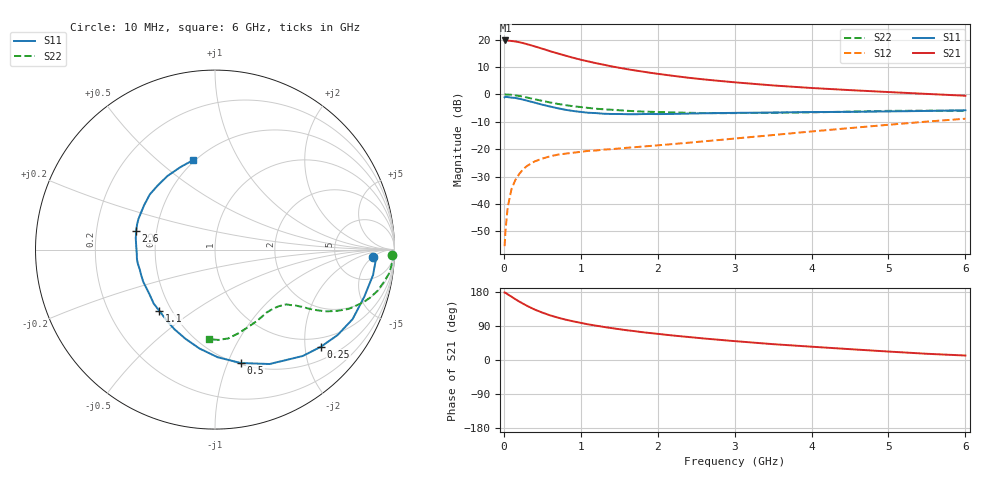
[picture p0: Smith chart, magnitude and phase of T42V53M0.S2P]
! Infineon Technologies  Discrete & RF Semiconductors
! BFR182T
! Si NPN RF Bipolar Junction Transistor in SC75
! VCE = 2.5 V  IC = 3 mA
! Common Emitter S-Parameters:  October  1999
# GHz  S  MA  R  50
!  f  S11  S21  S12  S22
! GHz  MAG  ANG  MAG  ANG  MAG  ANG  MAG  ANG
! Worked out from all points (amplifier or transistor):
!   36 points, 10 MHz to 6 GHz, reference 50 ohm
!   highest |S21| = 19.7 dB at 20 MHz (marker M1)
!   |S21| within 3 dB of that: start of sweep to 498.4 MHz
!   unconditionally stable (mu >= 1): 1.693 GHz to 4.2 GHz
!   at 250 MHz: K = 0.19, MSG = 23.0 dB, |S12| = -27.4 dB
!   at 1.4 GHz: K = 0.90, MSG = 15.1 dB, |S12| = -20.0 dB
!   at 6 GHz: K = 0.83, MSG = 4.2 dB, |S12| = -8.9 dB
!   lowest NFmin = 1.10 dB at 450 MHz
!   S11 on the Smith chart (normalised r, x): 10 MHz: 14, -6; 250 MHz: 0.78, -2.35; 500 MHz: 0.51, -1.12; 1.1 GHz: 0.43, -0.37; 2.6 GHz: 0.38, +0.10; 6 GHz: 0.49, +0.66
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0.01  0.8841 -2.8  9.562 178.1  0.0017 74.5  0.9877 -1.6
0.02  0.9004 -2.3  9.624 177.6  0.0031 91.3  0.9968 -1.6
0.05  0.8919 -9.2  9.572 173.3  0.0087 88.1  0.9902 -3.9
0.1  0.872 -17.6  9.406 167.1  0.0188 81.3  0.9805 -7.6
0.15  0.859 -26.8  9.23 160.4  0.0274 75.8  0.9573 -11.0
0.2  0.8325 -34.9  8.951 154.3  0.0353 73.3  0.9345 -14.2
0.25  0.8008 -42.5  8.608 148.6  0.0428 67.9  0.9057 -17.1
0.3  0.7683 -50.5  8.25 143.1  0.0493 64.9  0.8771 -19.6
0.4  0.7063 -64.5  7.52 133.2  0.0598 58.8  0.8154 -23.9
0.5  0.6483 -77.1  6.802 125.1  0.0673 54.4  0.7602 -26.7
0.6  0.5998 -88.6  6.142 117.9  0.074 51.3  0.7119 -28.9
0.8  0.5231 -108.4  5.098 106.6  0.0829 47.6  0.6367 -31.6
0.9  0.4977 -117.1  4.658 102.1  0.086 46.8  0.607 -32.5
1.1  0.4613 -132.2  3.984 93.9  0.0931 45.7  0.5656 -34.0
1.3  0.4425 -145.2  3.47 87.3  0.0982 46.0  0.5336 -35.5
1.6  0.435 -161.3  2.886 78.5  0.106 47.4  0.5016 -37.5
2.2  0.4396 177.2  2.177 64.6  0.1241 51.9  0.4686 -43.4
2.6  0.4515 166.6  1.875 56.8  0.1391 54.8  0.4567 -48.2
3.5  0.466 148.1  1.454 41.8  0.1811 58.6  0.4613 -59.9
4.5  0.4792 131.7  1.195 28.6  0.2427 58.8  0.4838 -74.2
5.5  0.4982 112.8  1.019 16.4  0.3187 55.4  0.5036 -87.8
6  0.513 103.9  0.944 11.8  0.3592 52.1  0.5001 -93.9
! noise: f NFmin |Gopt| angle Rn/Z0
0.45  1.1  0.37  30  0.33
0.9  1.2  0.35  61  0.26
1.8  1.85  0.27  133  0.2
